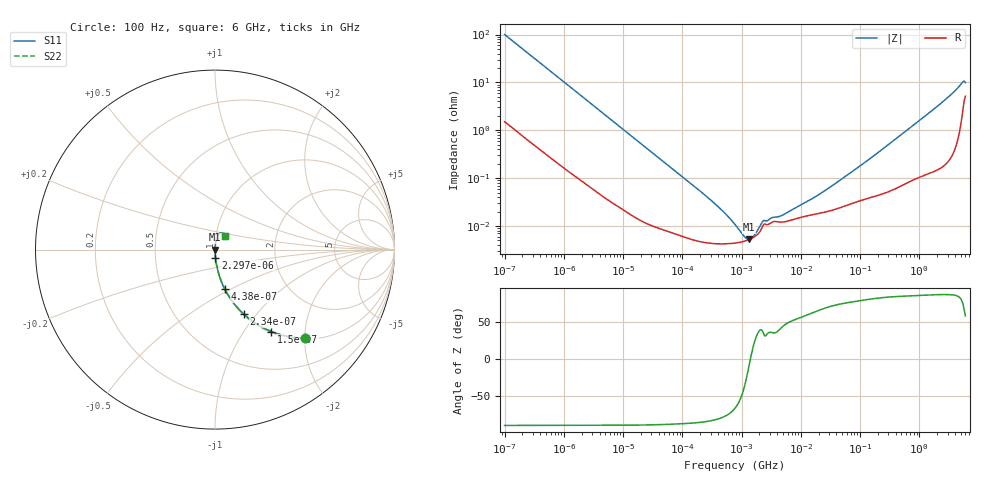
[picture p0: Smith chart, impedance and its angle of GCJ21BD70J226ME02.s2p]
!Murata Part Number: GCJ21BD70J226ME02
!These Parameters are Measured in Series Mode Connection
!Data Generated on Mar 13, 2026
!  o--ll--o
!Port1  Port2
!  o------o
!Operation Temp=25[degC], DC Bias Voltage=0[V]
!Freq. Start=100[Hz] Stop=6[GHz] 401[Steps]
# Hz S RI R 50
!Freq.(Hz) S11(Real) S11(Imag) S21(Real) S21(Imag) S12(Real) S12(Imag) S22(Real) S22(Imag)
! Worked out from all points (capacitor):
!   401 points, 100 Hz to 6 GHz, reference 50 ohm
!   read as one part in series: C = 15.8 uF near 109 Hz
!   lowest |Z| = 5.26 mohm at 1.326 MHz (marker M1)
!   series resonance near 1.404 MHz, so ESL is about 810 pH
!   S11 on the Smith chart (normalised r, x): 100 Hz: 1.03, -2.00; 150 Hz: 1.02, -1.35; 234 Hz: 1.01, -0.86; 438 Hz: 1.01, -0.46; 2.297 kHz: 1.00, -0.09; 6 GHz: 1.10, +0.17
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100  0.5011 -0.4925  0.4989 0.4925  0.4989 0.4925  0.5011 -0.4925
150  0.3143 -0.4567  0.6857 0.4567  0.6857 0.4567  0.3143 -0.4567
234  0.1609 -0.36  0.8391 0.36  0.8391 0.36  0.1609 -0.36
438  0.0542 -0.2188  0.9458 0.2188  0.9458 0.2188  0.0542 -0.2188
897  0.0146 -0.1123  0.9854 0.1123  0.9854 0.1123  0.0146 -0.1123
2008  0.00349 -0.0512  0.9965 0.0512  0.9965 0.0512  0.00349 -0.0512
2297  0.00278 -0.0449  0.9972 0.0449  0.9972 0.0449  0.00278 -0.0449
40335  9.61e-05 -0.00264  0.9999 0.00264  0.9999 0.00264  9.61e-05 -0.00264
302498  4.36e-05 -0.000345  1 0.000345  1 0.000345  4.36e-05 -0.000345
495019  4.24e-05 -0.000194  1 0.000194  1 0.000194  4.24e-05 -0.000194
774597  4.39e-05 -9.86e-05  1 9.86e-05  1 9.86e-05  4.39e-05 -9.86e-05
885955  4.51e-05 -7.46e-05  1 7.46e-05  1 7.46e-05  4.51e-05 -7.46e-05
1325623  5.18e-05 -9e-06  0.9999 9e-06  0.9999 9e-06  5.18e-05 -9e-06
1896632  6.85e-05 4.97e-05  0.9999 -4.97e-05  0.9999 -4.97e-05  6.85e-05 4.97e-05
2372521  0.000109 7.35e-05  0.9999 -7.35e-05  0.9999 -7.35e-05  0.000109 7.35e-05
4856642  0.000121 0.000116  0.9999 -0.000116  0.9999 -0.000116  0.000121 0.000116
1.555665e7  0.000172 0.000331  0.9998 -0.000331  0.9998 -0.000331  0.000172 0.000331
5.699437e7  0.000265 0.00106  0.9997 -0.00106  0.9997 -0.00106  0.000265 0.00106
3.124326e8  0.000556 0.00517  0.9994 -0.00517  0.9994 -0.00517  0.000556 0.00517
2.34314e9  0.003 0.0368  0.997 -0.0368  0.997 -0.0368  0.003 0.0368
5.245841e9  0.0272 0.0915  0.9728 -0.0915  0.9728 -0.0915  0.0272 0.0915
6e9  0.0548 0.0756  0.9452 -0.0756  0.9452 -0.0756  0.0548 0.0756
